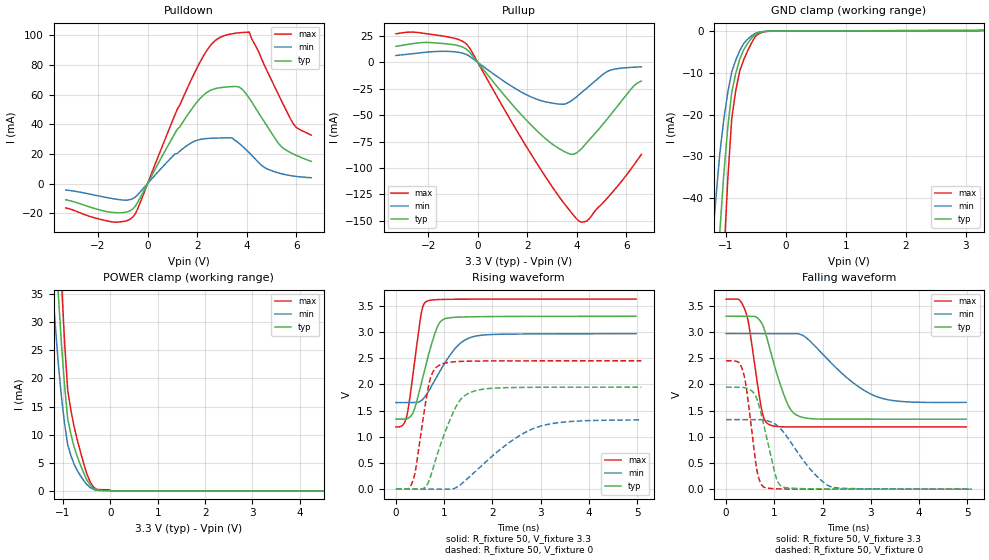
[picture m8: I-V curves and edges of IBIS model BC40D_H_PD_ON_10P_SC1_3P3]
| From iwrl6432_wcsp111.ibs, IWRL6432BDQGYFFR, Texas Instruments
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|   Model Cell BC40D_H_PD_ON_10P_SC1_3P3
|BC40D_H_PD_ON_10P_SC1_3P3
[Model]   BC40D_H_PD_ON_10P_SC1_3P3
Model_type   I/O
Polarity   Non-Inverting
Enable   Active-Low
Vinl =  0.8V
Vinh =  2V
Cref =  15pF
Rref =  100.0000M
Vref =  0V
Vmeas =  1.65
C_comp   2.157014p   1.997104p   2.250886p
|[Input load] weak_pd_on
|[Output drive] slow
|[supplytol] 10
|[temp] ind
[Model Spec]
Vinl   0.8V   0.8V   0.8V
Vinh   2V   2V   2V
[Temperature Range]   25   125   -40
[Voltage Range]   3.3   2.97   3.63
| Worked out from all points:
|   slope of the pulldown table from 0 to 0.495 V, typ, clamps not added: 31.8 ohm
|   slope of the pullup table from 0 to 0.495 V, typ, clamps not added: 33.8 ohm
|   GND clamp passes 1 mA (typ) near -0.52 V on its own axis
|   POWER clamp passes 1 mA (typ) near -0.42 V on its own axis
|   rising waveform, R_fixture 50, V_fixture 3.3: 20-80 % time 338ps typ, 538ps min, 211ps max; typ from 1.33 V to 3.3 V
|   rising waveform, R_fixture 50, V_fixture 0: 20-80 % time 469ps typ, 1.07ns min, 245ps max; typ from 0 V to 1.95 V
|   falling waveform, R_fixture 50, V_fixture 3.3: 20-80 % time 388ps typ, 937ps min, 235ps max; typ from 3.3 V to 1.33 V
|   falling waveform, R_fixture 50, V_fixture 0: 20-80 % time 295ps typ, 648ps min, 201ps max; typ from 1.95 V to 0 V
| Nom Voltages:
|   VDD=1.1001, VDDS=3.3, VDDS18=1.8, ESD_BIASFET=0, VSS=0, VSSS=0
| Min Voltages:
|   VDD=0.99, VDDS=2.97, VDDS18=1.62, ESD_BIASFET=0, VSS=0, VSSS=0
| Max Voltages:
|   VDD=1.21, VDDS=3.63, VDDS18=1.98, ESD_BIASFET=0, VSS=0, VSSS=0
[POWER_clamp]
|   voltage   I(typ)   I(min)   I(max)
-3.3V     446.9mA    419.5mA    603.9mA
-1.233V   56.59mA    37.53mA    80.37mA
-1.167V   45.68mA    29.91mA    65.17mA
-1.1V     35.14mA    22.67mA    50.36mA
-1.033V   26.13mA    16.78mA    37.31mA
-966.7mV  18.67mA    11.95mA    26.46mA
-900mV    12.76mA    8.172mA    17.82mA
-833.3mV  10.07mA    6.29mA     14.35mA
-566.7mV  3.276mA    1.904mA    4.983mA
-366.7mV  519.9uA    307.2uA    792.3uA
33.33mV   0A         0A         0A
6.6V      0A         0A         0A
[Pulldown]
|   voltage   I(typ)   I(min)   I(max)
-3.3V     -10.93mA   -4.311mA   -16.48mA
-1.4V     -19.53mA   -10.23mA   -25.96mA
-600mV    -17.23mA   -10.26mA   -22.66mA
1.1V      33.82mA    19.89mA    46.25mA
2V        55.14mA    29.24mA    78.29mA
2.6V      63.35mA    30.61mA    94.44mA
3.2V      65.21mA    30.81mA    100.4mA
3.7V      65.09mA    27.02mA    101.8mA
4.1V      57.64mA    20.71mA    102.2mA
5.3V      26.68mA    7.058mA    59.31mA
5.9V      19.77mA    5.007mA    39.76mA
6.6V      14.97mA    3.923mA    32.7mA
[Pullup]
|   voltage   I(typ)   I(min)   I(max)
-3.3V     15.12mA    6.498mA    27.02mA
-1.9V     18.73mA    9.943mA    26.53mA
-900mV    16.4mA     9.888mA    22.58mA
-400mV    11.39mA    6.786mA    15.98mA
2.4V      -65.08mA   -35.06mA   -96.18mA
3.5V      -84.52mA   -39.53mA   -134mA
3.8V      -87.17mA   -36.01mA   -143mA
4.1V      -83.69mA   -30.35mA   -150.6mA
4.4V      -75.99mA   -24.42mA   -150.3mA
5.3V      -51.41mA   -7.872mA   -126.6mA
6.3V      -22.29mA   -4.606mA   -97.15mA
6.6V      -17.71mA   -4.277mA   -87.2mA
[GND_clamp]
|   voltage   I(typ)   I(min)   I(max)
-3.3V     -787.2mA   -607.8mA   -1.235A
-1.233V   -85.66mA   -52.14mA   -138.8mA
-1.167V   -66.47mA   -40.37mA   -107.7mA
-1.1V     -48.25mA   -29.37mA   -77.99mA
-1.033V   -34.28mA   -21.19mA   -54.56mA
-966.7mV  -23.07mA   -14.67mA   -35.51mA
-900mV    -14.62mA   -9.792mA   -20.84mA
-833.3mV  -10.07mA   -6.938mA   -14.17mA
-700mV    -4.435mA   -2.939mA   -6.836mA
-500mV    -641.2uA   -454.5uA   -1.12mA
-300mV    -31.62uA   -32.73uA   -44.27uA
3.3V      108.6uA    159.4uA    198.5uA
[Ramp]
| variable   typ   min   max
dV/dt_f  1.1800166/0.38879804n 0.79472941/0.94541502n  1.4664299/0.23530429n
dV/dt_r  1.1731217/0.47024374n 0.80241661/1.0827371n  1.4753454/0.24601194n
R_load = 50
[Rising Waveform]
R_fixture = 50
V_fixture = 3.3
V_fixture_min = 2.97
V_fixture_max = 3.63
|   time   V(typ)   V(min)   V(max)
0s        1.335V     1.651V     1.187V
145.8ps   1.335V     1.651V     1.226V
223.5ps   1.342V     1.651V     1.388V
363.3ps   1.477V     1.651V     2.258V
518.8ps   1.994V     1.685V     3.321V
632ps     2.413V     1.804V     3.581V
927.7ps   3.2V       2.277V     3.619V
1.259ns   3.281V     2.718V     3.624V
1.575ns   3.289V     2.903V     3.625V
4.974ns   3.298V     2.966V     3.627V
[Rising Waveform]
R_fixture = 50
V_fixture = 0
V_fixture_min = 0
V_fixture_max = 0
|   time   V(typ)   V(min)   V(max)
0s        0V         0V         0V
251.4ps   0V         0V         0V
352.4ps   0V         0V         159.1mV
564.3ps   10.44mV    0V         1.355V
692.5ps   176mV      0V         2.041V
909.7ps   810.6mV    0V         2.37V
1.284ns   1.638V     50.3mV     2.435V
1.63ns    1.873V     326.1mV    2.444V
2.951ns   1.944V     1.19V      2.449V
5.084ns   1.946V     1.321V     2.449V
[Falling Waveform]
R_fixture = 50
V_fixture = 3.3
V_fixture_min = 2.97
V_fixture_max = 3.63
|   time   V(typ)   V(min)   V(max)
0s        3.298V     2.968V     3.626V
266.2ps   3.298V     2.968V     3.616V
409.5ps   3.298V     2.968V     3.376V
486.9ps   3.298V     2.968V     3.054V
738.2ps   3.166V     2.968V     1.515V
886.8ps   2.748V     2.968V     1.235V
1.252ns   1.673V     2.968V     1.188V
1.522ns   1.387V     2.956V     1.187V
3.084ns   1.335V     1.778V     1.186V
4.974ns   1.334V     1.654V     1.186V
[Falling Waveform]
R_fixture = 50
V_fixture = 0
V_fixture_min = 0
V_fixture_max = 0
|   time   V(typ)   V(min)   V(max)
0s        1.945V     1.327V     2.448V
250.2ps   1.945V     1.327V     2.426V
350.9ps   1.941V     1.327V     2.247V
427.2ps   1.925V     1.327V     1.891V
642.5ps   1.712V     1.327V     346.9mV
785.7ps   1.208V     1.319V     37.41mV
1.034ns   232mV      1.231V     6.916mV
1.189ns   37.94mV    1.09V      3.359mV
2.18ns    3.041mV    43.91mV    0V
5.084ns   0V         0V         0V
